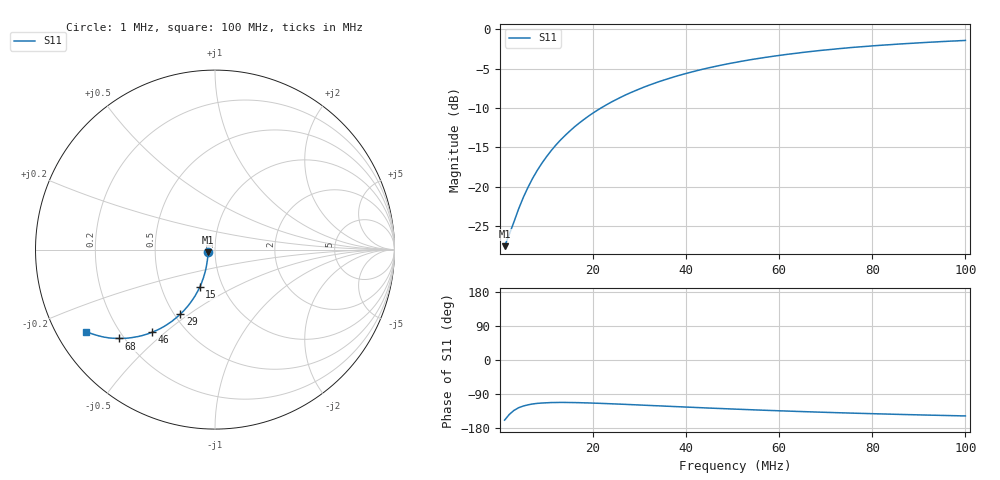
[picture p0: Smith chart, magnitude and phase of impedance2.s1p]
# Hz S RI R 50.0
! written by SimSmith version 18.3b
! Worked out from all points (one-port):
!   100 points, 1 MHz to 100 MHz, reference 50 ohm
!   lowest |S11| = -27.6 dB at 1 MHz (marker M1), VSWR 1.09, Z = 46.2 - j1.42 ohm
!   |S11| at or under -10 dB: start of sweep to 21.67 MHz
!   S11 on the Smith chart (normalised r, x): 1 MHz: 0.92, -0.03; 15 MHz: 0.78, -0.34; 29 MHz: 0.54, -0.46; 46 MHz: 0.33, -0.45; 68 MHz: 0.18, -0.38; 100 MHz: 0.09, -0.29
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1000000  -0.039 -0.0153
2000000  -0.0401 -0.0295
3000000  -0.0408 -0.0436
4000000  -0.0424 -0.0584
5000000  -0.0446 -0.0727
6000000  -0.047 -0.0869
7000000  -0.0496 -0.1013
8000000  -0.0526 -0.1155
9000000  -0.0564 -0.1292
1e7  -0.0605 -0.1429
1.2e7  -0.0695 -0.1703
1.4e7  -0.0794 -0.1965
1.5e7  -0.0854 -0.2091
1.7e7  -0.0976 -0.2342
2e7  -0.1185 -0.2695
2.3e7  -0.1414 -0.302
2.6e7  -0.1664 -0.3319
2.9e7  -0.1924 -0.3588
3.4e7  -0.2383 -0.3982
3.9e7  -0.2855 -0.4292
4.6e7  -0.3519 -0.4609
5.1e7  -0.3978 -0.4763
5.5e7  -0.4331 -0.4852
6.3e7  -0.4989 -0.4941
6.8e7  -0.5374 -0.4952
7.6e7  -0.5924 -0.4918
8.8e7  -0.6616 -0.4766
1e8  -0.7187 -0.4565
